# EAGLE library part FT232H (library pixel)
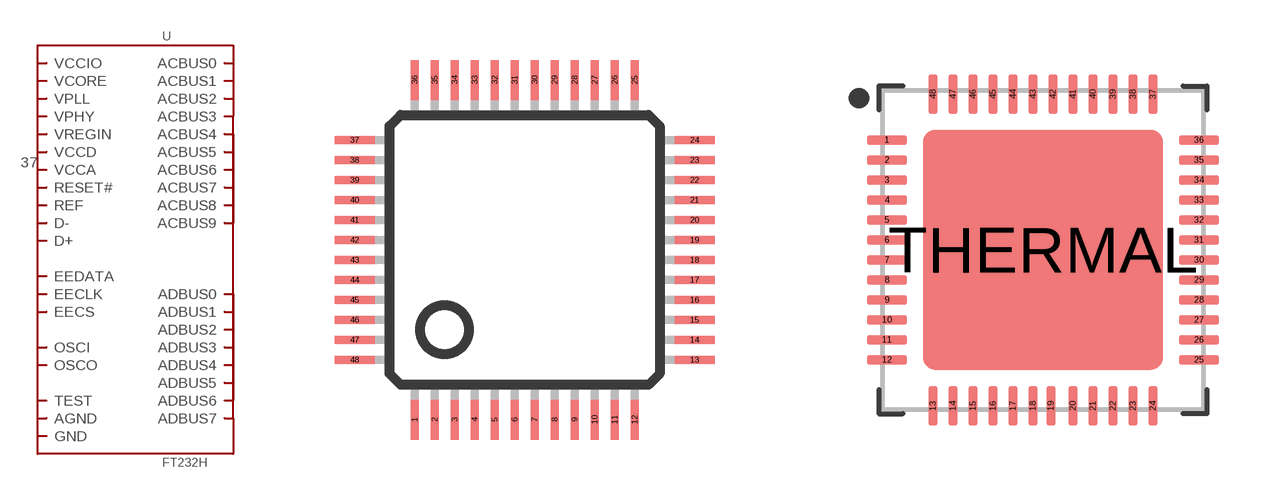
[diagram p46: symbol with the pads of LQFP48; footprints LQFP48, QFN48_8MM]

Designator prefix -

## FT232H  [LQFP48]
1  OSCI
2  OSCO
3  VPHY
4  AGND
5  REF
6  D-
7  D+
8  VPLL
9  AGND
10  GND
11  GND
12  VCCIO
13  ADBUS0
14  ADBUS1
15  ADBUS2
16  ADBUS3
17  ADBUS4
18  ADBUS5
19  ADBUS6
20  ADBUS7
21  ACBUS0
22  GND
23  GND
24  VCCIO
25  ACBUS1
26  ACBUS2
27  ACBUS3
28  ACBUS4
29  ACBUS5
30  ACBUS6
31  ACBUS7
32  ACBUS8
33  ACBUS9
34  RESET#
35  GND
36  GND
37  VCCA
38  VCORE
39  VCCD
40  VREGIN
41  AGND
42  TEST
43  EEDATA
44  EECLK
45  EECS
46  VCCIO
47  GND
48  GND

## FT232HQFN  [QFN48_8MM]
1  OSCI
2  OSCO
3  VPHY
4  AGND
5  REF
6  D-
7  D+
8  VPLL
9  AGND
10  GND
11  GND
12  VCCIO
13  ADBUS0
14  ADBUS1
15  ADBUS2
16  ADBUS3
17  ADBUS4
18  ADBUS5
19  ADBUS6
20  ADBUS7
21  ACBUS0
22  GND
23  GND
24  VCCIO
25  ACBUS1
26  ACBUS2
27  ACBUS3
28  ACBUS4
29  ACBUS5
30  ACBUS6
31  ACBUS7
32  ACBUS8
33  ACBUS9
34  RESET#
35  GND
36  GND
37  VCCA
38  VCORE
39  VCCD
40  VREGIN
41  AGND
42  TEST
43  EEDATA
44  EECLK
45  EECS
46  VCCIO
47  GND
48  GND
THERMAL  GND

## Footprint LQFP48 (pad centres in mm)
48-pin plastic LQFP (FPT-48P-M26) www.fma.fujitsu.com/pdf/e713717.pdf
smd 0.2 x 1: 1 -2.75,-4.25; 2 -2.25,-4.25; 3 -1.75,-4.25; 4 -1.25,-4.25; 5 -0.75,-4.25; 6 -0.25,-4.25; 7 0.25,-4.25; 8 0.75,-4.25; 9 1.25,-4.25; 10 1.75,-4.25; 11 2.25,-4.25; 12 2.75,-4.25; 25 2.75,4.25; 26 2.25,4.25; 27 1.75,4.25; 28 1.25,4.25; 29 0.75,4.25; 30 0.25,4.25; 31 -0.25,4.25; 32 -0.75,4.25; 33 -1.25,4.25; 34 -1.75,4.25; 35 -2.25,4.25; 36 -2.75,4.25
smd 1 x 0.2: 13 4.25,-2.75; 14 4.25,-2.25; 15 4.25,-1.75; 16 4.25,-1.25; 17 4.25,-0.75; 18 4.25,-0.25; 19 4.25,0.25; 20 4.25,0.75; 21 4.25,1.25; 22 4.25,1.75; 23 4.25,2.25; 24 4.25,2.75; 37 -4.25,2.75; 38 -4.25,2.25; 39 -4.25,1.75; 40 -4.25,1.25; 41 -4.25,0.75; 42 -4.25,0.25; 43 -4.25,-0.25; 44 -4.25,-0.75; 45 -4.25,-1.25; 46 -4.25,-1.75; 47 -4.25,-2.25; 48 -4.25,-2.75

## Footprint QFN48_8MM (pad centres in mm)
smd 1 x 0.23: 1 -3.9,2.75; 2 -3.9,2.25; 3 -3.9,1.75; 4 -3.9,1.25; 5 -3.9,0.75; 6 -3.9,0.25; 7 -3.9,-0.25; 8 -3.9,-0.75; 9 -3.9,-1.25; 10 -3.9,-1.75; 11 -3.9,-2.25; 12 -3.9,-2.75; 25 3.9,-2.75; 26 3.9,-2.25; 27 3.9,-1.75; 28 3.9,-1.25; 29 3.9,-0.75; 30 3.9,-0.25; 31 3.9,0.25; 32 3.9,0.75; 33 3.9,1.25; 34 3.9,1.75; 35 3.9,2.25; 36 3.9,2.75
smd 0.23 x 1: 13 -2.75,-3.9; 14 -2.25,-3.9; 15 -1.75,-3.9; 16 -1.25,-3.9; 17 -0.75,-3.9; 18 -0.25,-3.9; 19 0.2,-3.9; 20 0.75,-3.9; 21 1.25,-3.9; 22 1.75,-3.9; 23 2.25,-3.9; 24 2.75,-3.9; 37 2.75,3.9; 38 2.25,3.9; 39 1.75,3.9; 40 1.25,3.9; 41 0.75,3.9; 42 0.25,3.9; 43 -0.25,3.9; 44 -0.75,3.9; 45 -1.25,3.9; 46 -1.75,3.9; 47 -2.25,3.9; 48 -2.75,3.9
smd 6 x 6: THERMAL 0,0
